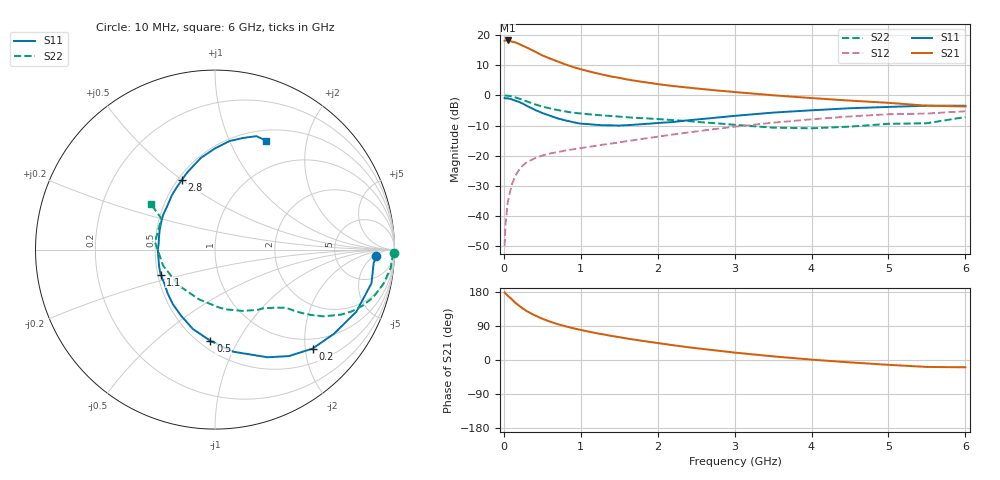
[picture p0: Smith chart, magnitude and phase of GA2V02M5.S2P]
! Infineon Technologies  Discrete & RF Semiconductors
! BF775
! Si NPN RF Bipolar Junction Transistor in SOT23
! VCE = 2 V  IC = 2.5 mA
! Common Emitter S-Parameters:  May  1996
# GHz  S  MA  R  50
!  f  S11  S21  S12  S22
! GHz  MAG  ANG  MAG  ANG  MAG  ANG  MAG  ANG
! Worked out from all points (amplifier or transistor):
!   36 points, 10 MHz to 6 GHz, reference 50 ohm
!   highest |S21| = 18.1 dB at 50 MHz (marker M1)
!   |S21| within 3 dB of that: start of sweep to 351.3 MHz
!   unconditionally stable (mu >= 1): 1.024 GHz to 4.246 GHz; 5.099 GHz to end of sweep
!   at 250 MHz: K = 0.32, MSG = 19.7 dB, |S12| = -23.1 dB
!   at 1.4 GHz: K = 1.13, MAG = 8.9 dB, |S12| = -16.0 dB
!   at 6 GHz: K = 1.01, MAG = 0.1 dB, |S12| = -5.3 dB
!   S11 on the Smith chart (normalised r, x): 10 MHz: 16, -6; 200 MHz: 0.78, -2.15; 500 MHz: 0.57, -0.78; 1.1 GHz: 0.52, -0.16; 2.8 GHz: 0.52, +0.50; 6 GHz: 0.63, +1.38
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0.01  0.8988 -2.4  7.964 178.3  0.0032 89.0  0.9954 -1.1
0.02  0.8871 -4.9  8.036 175.9  0.0068 84.0  0.9895 -2.4
0.05  0.8918 -12.1  8.055 170.1  0.0168 82.6  0.9842 -6.0
0.1  0.8603 -23.7  7.74 160.9  0.0324 76.8  0.9579 -11.4
0.15  0.8116 -35.4  7.472 150.9  0.0469 70.2  0.9218 -16.7
0.2  0.7743 -45.4  7.022 143.0  0.0592 65.3  0.8788 -20.9
0.25  0.7225 -55.2  6.546 135.6  0.0698 60.8  0.835 -24.4
0.3  0.6675 -64.0  6.137 128.7  0.0783 57.4  0.7916 -27.2
0.4  0.5778 -79.9  5.318 118.2  0.0905 52.2  0.7115 -31.5
0.5  0.5089 -92.9  4.554 108.9  0.1007 48.8  0.6505 -34.1
0.6  0.4591 -105.6  4.044 101.3  0.1089 46.9  0.6067 -35.8
0.7  0.4141 -117.1  3.62 94.7  0.1152 45.7  0.5696 -37.3
0.8  0.3846 -127.6  3.238 89.0  0.1218 45.2  0.5395 -38.3
0.9  0.3594 -137.2  2.936 83.9  0.1278 45.2  0.5153 -39.2
1.1  0.3334 -155.4  2.497 75.1  0.1401 45.2  0.4859 -41.8
1.6  0.3201 167.2  1.828 56.6  0.1742 46.4  0.4335 -48.7
2.2  0.3613 136.9  1.421 39.0  0.2247 46.1  0.3882 -60.9
2.8  0.4311 115.1  1.19 24.2  0.2818 42.6  0.3413 -78.2
3.5  0.5169 98.8  0.999 9.6  0.3518 35.8  0.2914 -107.8
4.5  0.6102 82.4  0.816 -6.3  0.447 23.3  0.3029 -162.9
5.5  0.6726 70.0  0.671 -18.3  0.4987 8.2  0.3447 150.0
6  0.6707 64.7  0.653 -19.3  0.5438 4.0  0.4365 144.6
